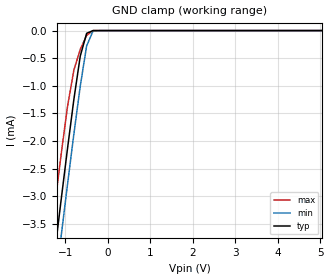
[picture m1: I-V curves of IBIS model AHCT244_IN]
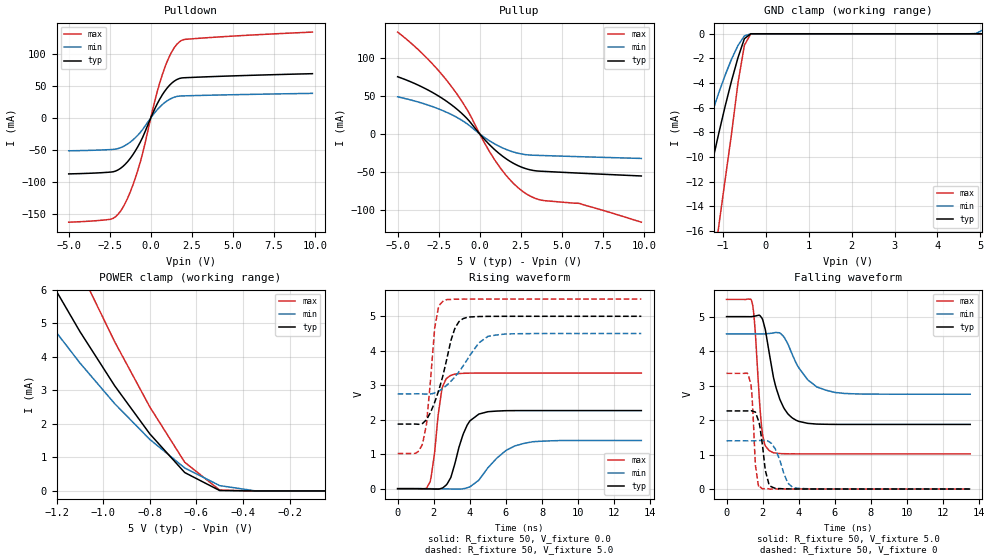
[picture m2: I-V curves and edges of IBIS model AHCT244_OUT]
| TEXAS INSTRUMENTS INCORPORATED
| Standard Linear and Logic Group
| IBIS Model of SN74AHCT244
| Octal Buffers/Drivers with 3-State Outputs
|  SOIC 20-pin (DW) package as [Component] AHCT244_DW
|  SSOP 20-pin (DB) package as [Component] AHCT244_DB
|  TVSOP 20-pin (DGV) package as [Component] AHCT244_DGV
|  TSSOP 20-pin (PW) package as [Component] AHCT244_PW
|  PDIP 20-pin (N) package as [Component] AHCT244_N
[IBIS Ver]   3.2
[Comment char]  |_char
[File Name]   ahct244.ibs
[File Rev]   1.1 | b_die
[Date]   September 11, 2000
[Source]   Data created from TI-SPICE simulations at TI-SLL.
[Notes]   The following is an IBIS list for the AHCT244.
   Please contact sllibis@ti.com with questions and
   comments concerning SLL IBIS models.
   These are the notes for the LVC244f.  Enter information on
   the warnings and plots.
   -As the input and output enable models are electrically
   same, we have used only one model for them
   -To comply with the data sheet we omitted the Vref
   and Rref from the Output Model
   -As there is no power clamp diode in the Input Model,
   we removed the Pwr Clamp table data from the Input Model
[Disclaimer] Property of Texas Instruments Incorporated.  Unauthorized
   reproduction and/or distribution is strictly prohibited.
   This product is protected under copyright law.
   Created  2000, (C) Copyright  2000, Texas Instruments Inc.,
   All Rights Reserved
   UNLESS THERE IS A SIGNED, WRITTEN AGREEMENT TO THE
   CONTRARY, TEXAS INSTRUMENTS (TI) IS PROVIDING THE IBIS
   MODELS  AND WITHOUT ANY WARRANTY, EXPRESSED OR
   IMPLIED.  TI assumes no liability for:
   1) the accuracy of the IBIS models provided to your
   company;
   2) the proper functioning of these IBIS Models in your
   design or for any resulting applications; or
   3) infringement of patents, copyrights or intellectual
   property rights resulting from your use of these IBIS
   models.
   TI provides IBIS Models as a service to our customers.
   You and your company shall not distribute, sell or give
   these models to anyone else without prior written
   permission from TI.
   TI reserves the right to make changes to our products or
   to discontinue any semiconductor product or service
   without notice, and advises our customers to obtain the
   latest version of relevant information to verify, before
   placing orders, that the information being relied on is
   current.
   Please be aware that your receipt and use of the IBIS
   information provided shall serve as acceptance of these
   terms and conditions.  If you do not accept these terms,
   you should return or destroy the IBIS models and any
   other accompanying information immediately.
| Component AHCT244_PW 20-pin TSSOP
[Component]   AHCT244_PW
[Manufacturer]   Texas Instruments, Inc.
[Package]
|   typ   min   max
R_pkg   3.500e-02   2.400e-02   4.700e-02
L_pkg   2.399e-09   1.710e-09   3.250e-09
C_pkg   2.840e-13   1.660e-13   4.180e-13
[Pin]   signal_name   model_name   R_pin   L_pin   C_pin
1   1OE_BAR   AHCT244_IN   4.100e-02   3.102e-09   4.100e-13
2   1A1   AHCT244_IN   4.000e-02   2.777e-09   3.630e-13
3   2Y4   AHCT244_OUT   2.900e-02   2.194e-09   2.600e-13
4   1A2   AHCT244_IN   2.500e-02   1.710e-09   1.660e-13
5   2Y3   AHCT244_OUT   2.500e-02   1.740e-09   1.910e-13
6   1A3   AHCT244_IN   2.400e-02   1.763e-09   1.930e-13
7   2Y2   AHCT244_OUT   2.400e-02   1.817e-09   1.740e-13
8   1A4   AHCT244_IN   2.800e-02   2.256e-09   2.650e-13
9   2Y1   AHCT244_OUT   4.500e-02   2.887e-09   3.680e-13
10   GND   GND   4.700e-02   3.250e-09   4.170e-13
11   2A1   AHCT244_IN   4.600e-02   3.244e-09   4.180e-13
12   1Y4   AHCT244_OUT   4.600e-02   2.961e-09   3.750e-13
13   2A2   AHCT244_IN   3.300e-02   2.334e-09   2.680e-13
14   1Y3   AHCT244_OUT   2.900e-02   1.915e-09   1.790e-13
15   2A3   AHCT244_IN   3.100e-02   1.934e-09   2.030e-13
16   1Y2   AHCT244_OUT   3.200e-02   1.917e-09   2.010e-13
17   2A4   AHCT244_IN   3.000e-02   1.833e-09   1.730e-13
18   1Y1   AHCT244_OUT   3.600e-02   2.324e-09   2.680e-13
19   2OE_BAR   AHCT244_IN   4.200e-02   2.869e-09   3.720e-13
20   VCC   POWER   4.200e-02   3.160e-09   4.140e-13
| Component AHCT244_DB 20-pin SSOP
[Component]   AHCT244_DB
[Manufacturer]   Texas Instruments, Inc.
[Package]
|   typ   min   max
R_pkg   0.04   0.035   0.051
L_pkg   3.495nH   3.035nH   4.314nH
C_pkg   0.42pF   0.346pF   0.502pF
[Pin]   signal_name   model_name   R_pin   L_pin   C_pin
1   1OE_BAR   AHCT244_IN   0.049   4.31nH   0.502pF
2   1A1   AHCT244_IN   0.048   3.903nH   0.487pF
3   2Y4   AHCT244_OUT  0.035   3.189nH   0.396pF
4   1A2   AHCT244_IN   0.035   3.036nH   0.347pF
5   2Y3   AHCT244_OUT  0.035   3.035nH   0.367pF
6   1A3   AHCT244_IN   0.035   3.035nH   0.367pF
7   2Y2   AHCT244_OUT  0.035   3.036nH   0.347pF
8   1A4   AHCT244_IN   0.035   3.189nH   0.397pF
9   2Y1   AHCT244_OUT  0.047   3.899nH   0.488pF
10   GND   GND   0.051   4.314nH   0.5pF
11   2A1   AHCT244_IN   0.051   4.314nH   0.5pF
12   1Y4   AHCT244_OUT  0.047   3.899nH   0.488pF
13   2A2   AHCT244_IN   0.035   3.189nH   0.397pF
14   1Y3   AHCT244_OUT  0.035   3.036nH   0.346pF
15   2A3   AHCT244_IN   0.035   3.035nH   0.367pF
16   1Y2   AHCT244_OUT  0.035   3.035nH   0.367pF
17   2A4   AHCT244_IN   0.035   3.036nH   0.346pF
18   1Y1   AHCT244_OUT  0.035   3.189nH   0.397pF
19   2OE_BAR   AHCT244_IN   0.047   3.899nH   0.488pF
20   VCC   POWER   0.051   4.314nH   0.502pF
| Component AHCT244_DW 20-pin SOIC
[Component]   AHCT244_DW
[Manufacturer]   Texas Instruments, Inc.
[Package]
|   typ   min   max
R_pkg   0.038   0.033   0.045
L_pkg   5.012nH   4.11nH   6.349nH
C_pkg   0.717pF   0.53pF   0.868pF
[Pin]   signal_name   model_name   R_pin   L_pin   C_pin
1   1OE_BAR   AHCT244_IN   0.042   6.336nH   0.865pF
2   1A1   AHCT244_IN   0.043   5.542nH   0.867pF
3   2Y4   AHCT244_OUT  0.034   4.714nH   0.732pF
4   1A2   AHCT244_IN   0.034   4.377nH   0.591pF
5   2Y3   AHCT244_OUT  0.036   4.13nH   0.533pF
6   1A3   AHCT244_IN   0.035   4.111nH   0.53pF
7   2Y2   AHCT244_OUT  0.034   4.284nH   0.583pF
8   1A4   AHCT244_IN   0.034   4.634nH   0.726pF
9   2Y1   AHCT244_OUT  0.04   5.518nH   0.865pF
10   GND   GND   0.043   6.349nH   0.866pF
11   2A1   AHCT244_IN   0.041   6.281nH   0.861pF
12   1Y4   AHCT244_OUT  0.045   5.561nH   0.868pF
13   2A2   AHCT244_IN   0.033   4.778nH   0.742pF
14   1Y3   AHCT244_OUT  0.035   4.414nH   0.596pF
15   2A3   AHCT244_IN   0.035   4.11nH   0.533pF
16   1Y2   AHCT244_OUT  0.036   4.13nH   0.533pF
17   2A4   AHCT244_IN   0.034   4.377nH   0.591pF
18   1Y1   AHCT244_OUT  0.034   4.714nH   0.731pF
19   2OE_BAR   AHCT244_IN   0.043   5.569nH   0.868pF
20   VCC   POWER   0.042   6.308nH   0.864pF
| Component AHCT244_N 20-pin PDIP
[Component]   AHCT244_N
[Manufacturer]   Texas Instruments, Inc.
[Package]
|   typ   min   max
R_pkg   0.043   0.038   0.05
L_pkg   7.384nH   4.68nH   10.321nH
C_pkg   0.51pF   0.231pF   0.821pF
[Pin]   signal_name   model_name   R_pin   L_pin   C_pin
1   1OE_BAR   AHCT244_IN   0.042   9.427nH   0.81pF
2   1A1   AHCT244_IN   0.046   8.544nH   0.456pF
3   2Y4   AHCT244_OUT  0.048   7.163nH   0.435pF
4   1A2   AHCT244_IN   0.04   4.825nH   0.261pF
5   2Y3   AHCT244_OUT  0.04   5.284nH   0.648pF
6   1A3   AHCT244_IN   0.04   4.686nH   0.232pF
7   2Y2   AHCT244_OUT  0.04   6.359nH   0.489pF
8   1A4   AHCT244_IN   0.038   7.982nH   0.475pF
9   2Y1   AHCT244_OUT  0.043   9.403nH   0.475pF
10   GND   GND   0.05   10.321nH   0.805pF
11   2A1   AHCT244_IN   0.05   10.281nH   0.81pF
12   1Y4   AHCT244_OUT  0.043   9.383nH   0.477pF
13   2A2   AHCT244_IN   0.038   7.978nH   0.476pF
14   1Y3   AHCT244_OUT  0.04   6.302nH   0.492pF
15   2A3   AHCT244_IN   0.04   4.68nH   0.231pF
16   1Y2   AHCT244_OUT  0.04   5.284nH   0.648pF
17   2A4   AHCT244_IN   0.04   4.822nH   0.261pF
18   1Y1   AHCT244_OUT  0.047   7.118nH   0.439pF
19   2OE_BAR   AHCT244_IN   0.046   8.492nH   0.461pF
20   VCC   POWER   0.043   9.348nH   0.821pF
| Component AHCT244_DGV 20-pin TVSOP
[Component]   AHCT244_DGV
[Manufacturer]   Texas Instruments, Inc.
[Package]
|   typ   min   max
R_pkg   0.044   0.038   0.048
L_pkg   2.561nH   2.236nH   2.961nH
C_pkg   0.342pF   0.264pF   0.446pF
[Pin]   signal_name   model_name   R_pin   L_pin   C_pin
1   1OE_BAR   AHCT244_IN   0.044   2.935nH   0.417pF
2   1A1   AHCT244_IN   0.042   2.869nH   0.446pF
3   2Y4   AHCT244_OUT  0.043   2.399nH   0.316pF
4   1A2   AHCT244_IN   0.044   2.236nH   0.265pF
5   2Y3   AHCT244_OUT  0.046   2.278nH   0.264pF
6   1A3   AHCT244_IN   0.045   2.274nH   0.264pF
7   2Y2   AHCT244_OUT  0.044   2.285nH   0.269pF
8   1A4   AHCT244_IN   0.043   2.452nH   0.32pF
9   2Y1   AHCT244_OUT  0.044   2.9nH   0.446pF
10   GND   GND   0.044   2.961nH   0.418pF
11   2A1   AHCT244_IN   0.045   2.954nH   0.418pF
12   1Y4   AHCT244_OUT  0.042   2.847nH   0.443pF
13   2A2   AHCT244_IN   0.045   2.453nH   0.319pF
14   1Y3   AHCT244_OUT  0.045   2.297nH   0.269pF
15   2A3   AHCT244_IN   0.048   2.334nH   0.268pF
16   1Y2   AHCT244_OUT  0.048   2.335nH   0.267pF
17   2A4   AHCT244_IN   0.046   2.299nH   0.268pF
18   1Y1   AHCT244_OUT  0.046   2.457nH   0.32pF
19   2OE_BAR   AHCT244_IN   0.043   2.848nH   0.441pF
20   VCC   POWER   0.038   2.812nH   0.408pF
| Models and submodels in the file (2): AHCT244_IN (Input), AHCT244_OUT (3-state)
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| Model AHCT244_IN
[Model]   AHCT244_IN
Model_type  Input
Vinl =   0.8
Vinh =   2.0
| variable   typ   min   max
C_comp   2.15pF   1.18pF   6.45pF
[Temperature Range]   40   100   -40
| Ambient temperature   25   85   -40
[Voltage range]   5.0   4.5   5.5
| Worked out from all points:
|   GND clamp passes 1 mA (typ) near -0.75 V on its own axis
[GND Clamp]
| AHCT244_IN
|   Voltage   I(typ)   I(min)   I(max)
-5V       -28.65mA   -29.28mA   -27.83mA
-1.4V     -4.97mA    -5.633mA   -4.119mA
-1.25V    -4.011mA   -4.673mA   -3.168mA
-1.1V     -3.063mA   -3.722mA   -2.24mA
-950mV    -2.133mA   -2.784mA   -1.373mA
-800mV    -1.243mA   -1.87mA    -713.7uA
-650mV    -460.1uA   -1.003mA   -340.4uA
-500mV    -49.75uA   -277uA     -86.57uA
-350mV    -65.13nA   -9.073uA   -15.4nA
-200mV    -864pA     -89.44nA   -791.6pA
5.05V     2.194nA    3.944nA    1.59nA
| Model AHCT244_OUT
[Model]   AHCT244_OUT
Model_type  3-state
Enable   Active-Low
|Vref =   0.0
Cref =   50p
|Rref =   1k
Vmeas =   1.5
| variable   typ   min   max
C_comp   5.49pF   3.07pF   11.37pF
| C_pullup   5.68pF   3.68pF   9.20pF
| C_pulldown   6.55pF   3.07pF   11.37pF
| C_tri-state   4.23pF   3.21pF   8.70pF
[Temperature Range]   40   100   -40
| Ambient temperature   25   85   -40
[Voltage range]   5.0   4.5   5.5
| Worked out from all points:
|   slope of the pulldown table from 0 to 0.75 V, typ, clamps not added: 19.8 ohm
|   slope of the pullup table from 0 to 0.75 V, typ, clamps not added: 43 ohm
|   GND clamp passes 1 mA (typ) near -0.56 V on its own axis
|   POWER clamp passes 1 mA (typ) near -0.71 V on its own axis
|   rising waveform, R_fixture 50, V_fixture 0.0: 20-80 % time 806ps typ, 1.5ns min, 448ps max; typ from 0 V to 2.27 V
|   rising waveform, R_fixture 50, V_fixture 5.0: 20-80 % time 950ps typ, 1.47ns min, 436ps max; typ from 1.87 V to 5 V
|   falling waveform, R_fixture 50, V_fixture 5.0: 20-80 % time 814ps typ, 1.22ns min, 339ps max; typ from 5 V to 1.87 V
|   falling waveform, R_fixture 50, V_fixture 0: 20-80 % time 345ps typ, 572ps min, 195ps max; typ from 2.27 V to 0 V
[GND Clamp]
| AHCT244_OUT
|   Voltage   I(typ)   I(min)   I(max)
-5V       -81.07mA   -55.17mA   -133.7mA
-2.15V    -25.98mA   -16.98mA   -44.96mA
-2V       -23.26mA   -15.11mA   -40.56mA
-1.55V    -15.39mA   -9.713mA   -27.73mA
-1.1V     -8.113mA   -4.819mA   -15.67mA
-800mV    -3.826mA   -2.063mA   -8.121mA
-650mV    -1.946mA   -954.8uA   -4.007mA
-500mV    -401.3uA   -177.4uA   -930.4uA
-350mV    -86.56nA   -4.487uA   -154.5nA
4.75V     1.165nA    218.4nA    1.219nA
4.9V      1.264nA    19.63uA    1.379nA
5.05V     1.374nA    289uA      1.562nA
[POWER Clamp]
| AHCT244_OUT
|   Voltage   I(typ)   I(min)   I(max)
-5V       75.06mA    57.21mA    95.48mA
-1.4V     8.474mA    6.63mA     11.4mA
-1.25V    6.543mA    5.167mA    8.913mA
-1.1V     4.754mA    3.817mA    6.584mA
-950mV    3.128mA    2.597mA    4.439mA
-800mV    1.701mA    1.537mA    2.505mA
-650mV    547.3uA    684.4uA    853.8uA
-500mV    10.84uA    158.3uA    24.77uA
-350mV    75.21nA    4.649uA    96.59nA
-50mV     1.374nA    1.777nA    8.27nA
[Pulldown]
| AHCT244_OUT
|   Voltage   I(typ)   I(min)   I(max)
-5V       -87.68mA   -51.49mA   -163.3mA
-2.45V    -84.85mA   -49.57mA   -158.7mA
-2.15V    -83.3mA    -48.89mA   -154.9mA
-1.7V     -76.08mA   -45.08mA   -140.3mA
-1.25V    -63.38mA   -37.87mA   -116mA
-650mV    -38.49mA   -23.1mA    -70.17mA
250mV     14.54mA    8.48mA     27.08mA
700mV     36mA       20.78mA    67.52mA
1.3V      54.93mA    31.1mA     104.5mA
1.75V     61.77mA    34.21mA    119.2mA
2.95V     63.88mA    35.13mA    124.7mA
9.85V     69.25mA    38.41mA    134.4mA
[Pullup]
| AHCT244_OUT
|   Voltage   I(typ)   I(min)   I(max)
-5V       75.33mA    48.83mA    134.2mA
-3.35V    60.09mA    39.41mA    102.8mA
-1.85V    40.4mA     26.83mA    66.14mA
-800mV    20.84mA    13.81mA    33.01mA
250mV     -6.238mA   -4.018mA   -10.16mA
1V        -22.43mA   -14.23mA   -36.95mA
1.75V     -34.83mA   -21.65mA   -58.17mA
2.5V      -43.41mA   -26.28mA   -73.77mA
3.1V      -47.51mA   -27.96mA   -82.21mA
3.7V      -49.17mA   -28.43mA   -87.05mA
6.1V      -51.78mA   -30.06mA   -91.68mA
9.85V     -55.48mA   -32.36mA   -116.4mA
[Ramp]
| AHCT244_OUT
| variable   typ   min   max
dV/dt_r   1.3678E+00/8.1007E-10  8.4808E-01/1.5044E-09  2.0210E+00/4.4994E-10
dV/dt_f   1.9038E+00/8.1721E-10  1.0747E+00/1.2193E-09  2.6951E+00/3.3414E-10
R_load = 50
[Rising Waveform]
| AHCT244_OUT_33
R_fixture = 50
V_fixture = 0.0
V_fixture_min = 0.0
V_fixture_max = 0.0
L_fixture = 0.0
C_fixture = 0.0
|   Time   V(typ)   V(min)   V(max)
0s        0V         0V         0V
1.8ns     -8.256mV   -853.3uV   201.8mV
2.05ns    -12.31mV   -2.602mV   1.047V
2.45ns    13.79mV    -5.445mV   2.887V
2.9ns     281.7mV    -9.069mV   3.274V
3.85ns    1.841V     25.76mV    3.35V
4.5ns     2.164V     247.1mV    3.354V
6ns       2.263V     1.107V     3.355V
7ns       2.265V     1.314V     3.355V
13.5ns    2.265V     1.398V     3.355V
[Rising Waveform]
| AHCT244_OUT
R_fixture =   50
V_fixture =   5.0
V_fixture_min = 4.5
V_fixture_max = 5.5
L_fixture = 0.0
C_fixture = 0.0
|   Time   V(typ)   V(min)   V(max)
0s        1.874V     2.75V      1.019V
1.35ns    1.885V     2.749V     1.261V
1.6ns     2.002V     2.743V     1.874V
2.05ns    2.5V       2.778V     4.648V
2.25ns    2.807V     2.824V     5.228V
2.5ns     3.258V     2.908V     5.434V
3.15ns    4.618V     3.231V     5.497V
3.85ns    4.97V      3.739V     5.499V
5.5ns     4.999V     4.46V      5.5V
13.5ns    5V         4.5V       5.5V
[Falling Waveform]
| AHCT244_OUT
R_fixture =   50
V_fixture =   5.0
V_fixture_min = 4.5
V_fixture_max = 5.5
L_fixture = 0.0
C_fixture = 0.0
|   Time   V(typ)   V(min)   V(max)
0s        5V         4.5V       5.5V
1.4ns     5.001V     4.5V       5.446V
1.55ns    5.014V     4.499V     4.834V
1.95ns    4.965V     4.499V     1.773V
2.1ns     4.721V     4.501V     1.324V
2.35ns    3.991V     4.511V     1.121V
2.95ns    2.604V     4.531V     1.029V
4ns       1.962V     3.517V     1.02V
6ns       1.874V     2.802V     1.019V
13.5ns    1.874V     2.75V      1.019V
[Falling Waveform]
| AHCT244_OUT
R_fixture = 50
V_fixture = 0
V_fixture_min = 0
V_fixture_max = 0
L_fixture = 0
C_fixture = 0
|   Time   V(typ)   V(min)   V(max)
0s        2.265V     1.398V     3.355V
1.15ns    2.265V     1.398V     3.36V
1.35ns    2.271V     1.397V     3.043V
1.6ns     2.231V     1.399V     692.4mV
1.8ns     1.935V     1.404V     41.06mV
2.15ns    535.9mV    1.405V     14.15mV
2.7ns     19.75mV    1.159V     5.654mV
3.4ns     4.344mV    169.5mV    -1.578mV
3.85ns    1.586mV    27.56mV    -1.061mV
13.5ns    187.2nV    169.9nV    5.11uV
